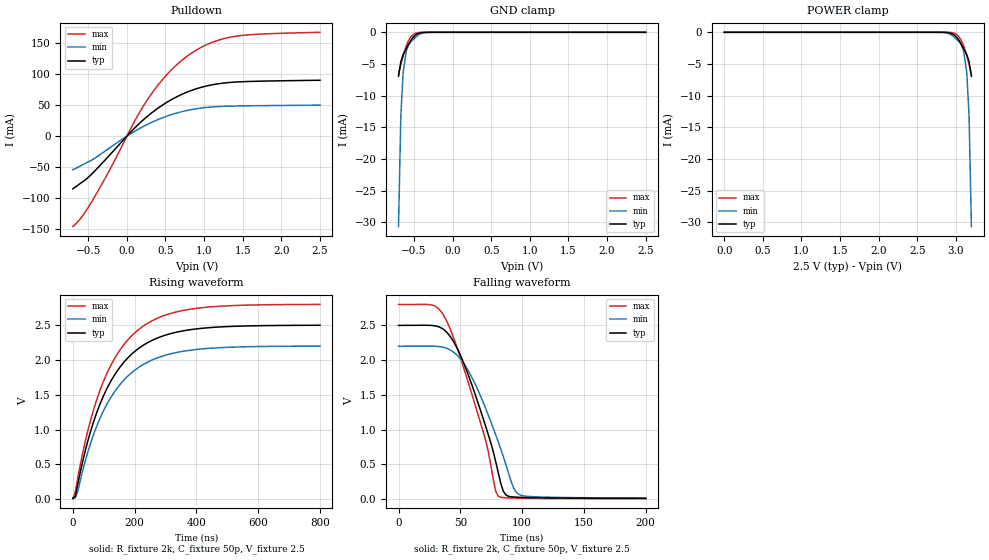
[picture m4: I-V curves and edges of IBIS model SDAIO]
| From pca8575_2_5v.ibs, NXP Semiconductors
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[Model]   SDAIO
Model_type I/O_open_drain
Enable Active-Low
Vinh=1.75
Vinl=0.75
Vref=2.5
Vmeas=1.25
Rref=2k
Cref=50p
C_comp   8p   7.8p   8.2p
[Temperature Range] 27   85   -40
[Voltage Range]   2.5   2.2   2.8
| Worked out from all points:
|   slope of the pulldown table from 0 to 0.375 V, typ, clamps not added: 8.8 ohm
|   GND clamp passes 1 mA (typ) near -0.52 V on its own axis
|   falling waveform, R_fixture 2k, C_fixture 50p, V_fixture 2.5: 20-80 % time 27.3ns typ, 28.6ns min, 27.7ns max; typ from 2.5 V to 0.01 V
|   rising waveform, R_fixture 2k, C_fixture 50p, V_fixture 2.5: 20-80 % time 142ns typ, 142ns min, 141ns max; typ from 0.009 V to 2.5 V
[Pulldown]
-700mV    -84.71mA   -54.07mA   -145.5mA
-570mV    -73.24mA   -46.02mA   -127.6mA
-440mV    -59.1mA    -37.35mA   -102.4mA
-220mV    -30.01mA   -18.56mA   -53.63mA
110mV     14.29mA    8.485mA    26.39mA
270mV     32.39mA    19.24mA    59.35mA
500mV     53.16mA    31.45mA    96.69mA
750mV     69.4mA     40.61mA    125.9mA
1.05V     81.35mA    46.49mA    148.2mA
1.34V     86.55mA    48.37mA    159.4mA
1.69V     88.45mA    49.07mA    164.1mA
2.5V      90.04mA    49.93mA    167.2mA
[GND Clamp]
-700mV    -6.935mA   -30.66mA   -6.593mA
-670mV    -4.642mA   -13.19mA   -5.083mA
-640mV    -3.526mA   -6.329mA   -3.662mA
-600mV    -2.591mA   -2.99mA    -2.148mA
-570mV    -1.922mA   -2.007mA   -1.319mA
-540mV    -1.276mA   -1.476mA   -736.2uA
-510mV    -783.4uA   -1.124mA   -364.6uA
-440mV    -172.9uA   -393.1uA   -38.38uA
-380mV    -28.35uA   -95.07uA   -3.19uA
-280mV    -665.7nA   -3.811uA   -30.99nA
2.5V      141pA      281.5pA    130.1pA
[POWER Clamp]
0V        141pA      281.5pA    130.1pA
2.78V     -665.7nA   -3.811uA   -30.99nA
2.88V     -28.35uA   -95.07uA   -3.19uA
2.94V     -172.9uA   -393.1uA   -38.38uA
3.01V     -783.4uA   -1.124mA   -364.6uA
3.04V     -1.276mA   -1.476mA   -736.2uA
3.07V     -1.922mA   -2.007mA   -1.319mA
3.1V      -2.591mA   -2.99mA    -2.148mA
3.14V     -3.526mA   -6.329mA   -3.662mA
3.17V     -4.642mA   -13.19mA   -5.083mA
3.2V      -6.935mA   -30.66mA   -6.593mA
[Falling Waveform]
R_fixture=2k
C_fixture=50p
V_fixture=2.5
V_fixture_min=2.2
V_fixture_max=2.8
0s        2.5V       2.2V       2.8V
28.28ns   2.497V     2.201V     2.787V
38.38ns   2.413V     2.175V     2.583V
56.57ns   1.782V     1.844V     1.672V
70.71ns   1.037V     1.296V     834.1mV
80.81ns   373.2mV    818.9mV    40.98mV
86.87ns   60.38mV    497.6mV    19.55mV
92.93ns   30.38mV    168.6mV    15.31mV
98.99ns   24.76mV    54.79mV    12.93mV
200ns     10.3mV     15.69mV    6.07mV
[Rising Waveform]
R_fixture=2k
C_fixture=50p
V_fixture=2.5
V_fixture_min=2.2
V_fixture_max=2.8
0s        9.182mV    13.6mV     5.538mV
8.081ns   34.25mV    20.09mV    99.54mV
16.16ns   215.9mV    111.8mV    304.3mV
48.48ns   832.7mV    673.3mV    980mV
96.97ns   1.461V     1.247V     1.667V
153.5ns   1.902V     1.651V     2.149V
218.2ns   2.182V     1.908V     2.455V
290.9ns   2.344V     2.056V     2.631V
396ns     2.444V     2.148V     2.74V
800ns     2.499V     2.199V     2.799V
[Ramp]
R_load=2k
dV/dt_r   1.494E+0/3.698E-9   1.491E+0/4.313E-9   1.497E+0/3.322E-9
dV/dt_f   1.494E+0/2.536E-8   1.489E+0/2.944E-8   1.497E+0/2.308E-8
|[End   SDAIO
